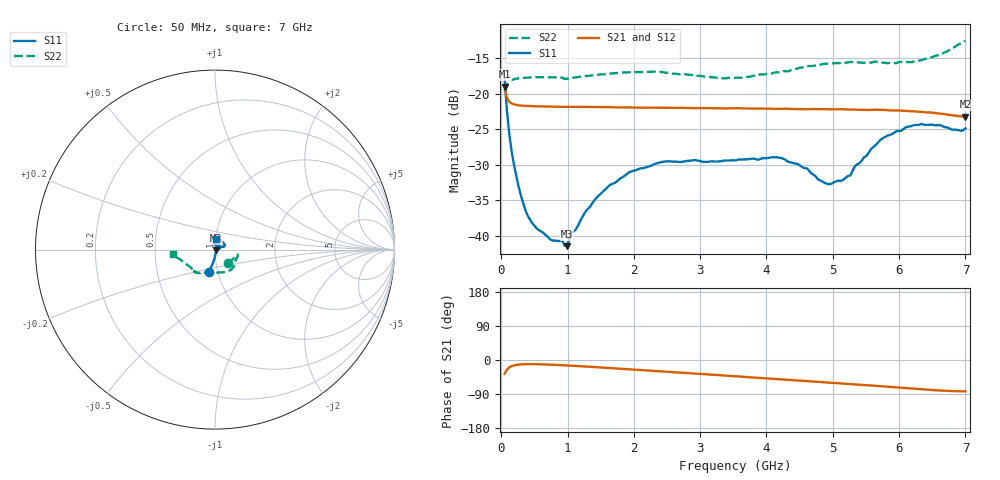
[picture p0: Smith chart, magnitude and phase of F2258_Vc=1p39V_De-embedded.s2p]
! Integrated Device Technology
! Corporate Headquarters
! 6024 Silver Creek Valley Road
! San Jose, CA 95138  USA
! Phone:  1-408-284-8200
! Toll Free:  1-800-223-1366
! Webpage:  http://www.idt.com/
! Timing and RF Division
! 515 Groton Road, Suite 102
! Westford, MA 01886-6024
! Device:  F2258
! Description: Voltage Variable RF Attenuator
! Frequency:  50.0 -  6000.00 MHz
! Package:  3x3 mm Thin QFN Plastic Package: 16 pin
! Ports:  2 RF, 2 DC
!  Pin  1  = NC
!  Pin  2  = NC
!  Pin  3  = RF2  = Port 2
!  Pin  4  = GND
!  Pin  5  = Vdd
!  Pin  6  = NC
!  Pin  7  = VCTRL
!  Pin  8  = NC
!  Pin  9  = GND
!  Pin 10  = RF1  = Port 1
!  Pin 11  = NC
!  Pin 12  = NC
!  Pin 13  = NC
!  Pin 14  = NC
!  Pin 15  = NC
!  Pin 16  = NC
! Vcntrl:  1.390 Volts
! Vdd:  +3.300 Volts
! Current:  1.161 mA
! Data:  The device was measured on a the F2258 evaluation board which has
!  individual transmission lines to the RF pins.  Data was collected
!  using a calibrated network analyzer.  The evaluation board was
!  de-embedded using a TRL calibration technique.
!  The reference plane is the edge of the package pin.
! Misc:  SN 10
!  Action Tracker AT0285
! Date Measured:  2014-12-10
! Date:  2016-01-13  MJV
! Note:
!  Integrated Device Technology supplies this data as a sample of measured
!  data at the package pin for this product.  Your particular data for this
!  product may vary.
!  Data was taken at 25 degrees C.
!  Integrated Device Technology reserves the right to change this data at anytime.
!Freq_(GHz)  S11M_(dB)  S11P_(deg)  S21M_(dB)  S21P_(deg)  S12M_(dB)  S12P_(deg)  S22M_(dB)  S22P_(deg)
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# GHz S dB R 50
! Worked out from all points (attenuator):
!   201 points, 50 MHz to 7 GHz, reference 50 ohm
!   highest |S21| = -18.96 dB at 50 MHz (marker M1); lowest = -23.2 dB at 7 GHz (marker M2)
!   lowest |S11| = -41.5 dB at 988.2 MHz (marker M3), VSWR 1.02, Z = 50.8 - j0.372 ohm
!   |S11| at or under -10 dB: start of sweep to end of sweep
!   |S22| runs from -19.6 to -12.5 dB; largest |S21 - S12| = 0.00061
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0.05  -17.89 -105.4  -18.96 -36.4  -18.96 -36.4  -19.58 -46.4
0.08475  -22.36 -98.6  -20.56 -25.4  -20.57 -25.4  -18.67 -23.4
0.15425  -28.01 -91.3  -21.34 -16.3  -21.35 -16.3  -18.04 -14.4
0.2585  -32.95 -81.9  -21.60 -12.1  -21.59 -12.1  -17.81 -12.1
0.36275  -36.34 -71.7  -21.69 -10.9  -21.69 -10.9  -17.72 -12.8
0.5365  -38.98 -52.0  -21.74 -11.0  -21.74 -11.0  -17.63 -15.4
0.98825  -41.46 -25.6  -21.82 -14.4  -21.81 -14.4  -17.86 -25.6
1.05775  -39.67 -16.2  -21.82 -15.0  -21.82 -15.0  -17.74 -26.9
1.2315  -37.19 -3.9  -21.83 -16.7  -21.83 -16.7  -17.51 -30.6
1.6485  -32.77 7.4  -21.87 -21.4  -21.87 -21.4  -17.13 -38.9
1.9265  -31.06 16.2  -21.91 -24.4  -21.91 -24.4  -16.96 -44.3
2.37825  -29.69 27.9  -21.95 -29.5  -21.96 -29.5  -16.91 -53.5
3.525  -29.37 80.7  -22.02 -42.9  -21.99 -43.0  -17.74 -90.7
4.22  -29.02 101.7  -22.11 -51.1  -22.11 -51.1  -16.89 -115.2
4.7065  -31.38 90.2  -22.13 -56.8  -22.11 -56.9  -16.05 -124.7
4.94975  -32.74 68.9  -22.18 -59.7  -22.17 -59.7  -15.74 -127.2
5.15825  -32.10 47.2  -22.18 -62.4  -22.19 -62.3  -15.63 -129.2
5.2625  -31.50 37.3  -22.21 -63.4  -22.20 -63.5  -15.49 -130.2
5.57525  -27.78 21.3  -22.25 -67.2  -22.23 -67.3  -15.59 -133.2
5.85325  -25.80 19.5  -22.32 -70.8  -22.32 -70.8  -15.64 -136.9
6.33975  -24.22 27.5  -22.55 -77.2  -22.54 -77.2  -15.24 -149.1
7  -24.84 83.7  -23.20 -82.7  -23.22 -82.6  -12.46 -173.8
